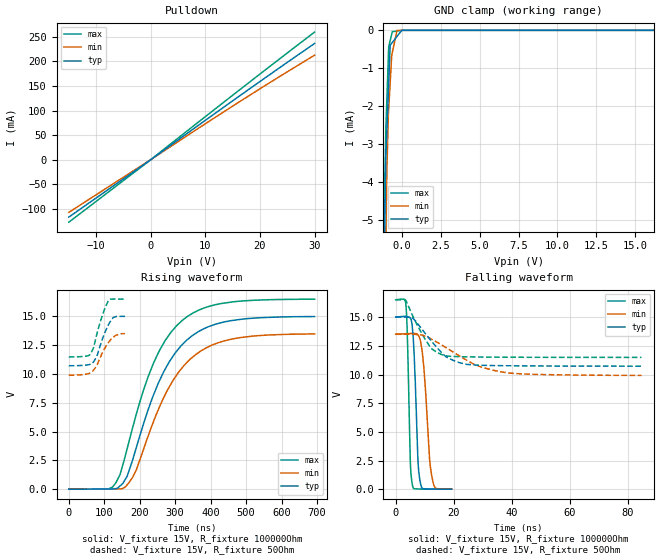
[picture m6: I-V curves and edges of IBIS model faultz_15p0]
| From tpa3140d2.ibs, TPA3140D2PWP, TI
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|   faultz_15p0 Model
[Model]   faultz_15p0
Model_type   Open_drain
Polarity   Non-Inverting
Vmeas = 7.5
Vref = 15
Cref = 2pF
Rref = 100000
|   typ   min   max
|   (nom PVT)   (fast PVT)   (slow PVT)
C_comp   1.652e-13   1.526e-13   1.894e-13
| Where nom  PVT is Nominal Process, 15V, 27C
|   Fast PVT is Strong Process,  16.5V, -40C
|   Slow PVT is Weak Process,   13.5V, 125C
[Voltage Range]   15   13.5   16.5
|Junction Temperature
[Temperature Range]   27   125   -40
[Pullup Reference]   15   13.5   16.5
[Pulldown Reference]   0   0   0
[Power Clamp Reference]   15   13.5   16.5
[GND Clamp Reference]   0   0   0
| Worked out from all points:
|   slope of the pulldown table from 0 to 2.25 V, typ, clamps not added: 124 ohm
|   GND clamp passes 1 mA (typ) near -0.82 V on its own axis
|   falling waveform, V_fixture 15V, R_fixture 100000Ohm: 20-80 % time 1.29ns typ, 2.03ns min, 919ps max; typ from 15 V to 0.026 V
|   rising waveform, V_fixture 15V, R_fixture 100000Ohm: 20-80 % time 120ns typ, 124ns min, 116ns max; typ from 0.019 V to 15 V
|   falling waveform, V_fixture 15V, R_fixture 50Ohm: 20-80 % time 8.71ns typ, 15.3ns min, 6.48ns max; typ from 15 V to 10.7 V
|   rising waveform, V_fixture 15V, R_fixture 50Ohm: 20-80 % time 30.6ns typ, 36.5ns min, 28ns max; typ from 10.7 V to 15 V
[Pulldown]
|   Voltage   I(typ)   I(min)   I(max)
-15V      -116.5mA   -106.9mA   -126.8mA
0V        0A         0A         0A
15.57V    124.1mA    112.9mA    135.8mA
30V       236.2mA    212.4mA    259.3mA
[GND Clamp]
|   Voltage   I(typ)   I(min)   I(max)
-15V      -1.129A    -780mA     -1.389A
-1.155V   -6.507mA   -9.239mA   -5.398mA
-1.121V   -5.497mA   -7.944mA   -4.25mA
-1.04V    -3.321mA   -5.528mA   -2.547mA
-972mV    -2.601mA   -3.62mA    -1.762mA
-858mV    -1.384mA   -2.064mA   -435.8uA
-765mV    -391.9uA   -1.386mA   -274.5uA
-675mV    -344.9uA   -729.4uA   -118.4uA
-627mV    -319.8uA   -587.6uA   -35.21uA
-324mV    -161.5uA   -1.414uA   -20.17uA
-15mV     0A         -65.47nA   -4.838uA
30V       0A         0A         0A
[POWER Clamp]
|   Voltage   I(typ)   I(min)   I(max)
-15V      0A         0A         0A
0V        0A         0A         0A
30V       0A         0A         0A
[Ramp]
R_load = 100000
|   typ   min   max
dV/dt_r   8.98683/1.20201e-07   8.08586/1.24554e-07   9.8876/1.15684e-07
dV/dt_f   8.98876/1.29126e-09   8.08874/2.02787e-09   9.88868/9.19156e-10
[Falling Waveform]
V_fixture = 15V
V_fixture_min = 13.5V
V_fixture_max = 16.5V
R_fixture = 100000Ohm
|   Time   V(typ)   V(min)   V(max)
0s        15V        13.5V      16.5V
3.485ns   15.06V     13.55V     16.18V
3.949ns   15.02V     13.55V     13.93V
5.121ns   14.87V     13.56V     1.914V
5.993ns   13.38V     13.57V     157.1mV
7.658ns   2.58V      13.44V     43.13mV
8.575ns   484mV      12.85V     37.44mV
11.66ns   37.6mV     2.647V     31.43mV
12.87ns   33.79mV    622.7mV    30.22mV
19.25ns   26.25mV    32.03mV    27.36mV
[Rising Waveform]
V_fixture = 15V
V_fixture_min = 13.5V
V_fixture_max = 16.5V
R_fixture = 100000Ohm
|   Time   V(typ)   V(min)   V(max)
0s        18.63mV    18.29mV    18.76mV
111.5ns   19.07mV    24.84mV    19.12mV
132.8ns   59.54mV    26.09mV    570.7mV
164.5ns   1.137V     382.9mV    3.516V
180.4ns   2.597V     1.053V     5.397V
239.5ns   8.232V     5.928V     10.99V
283.4ns   11.07V     8.883V     13.42V
319.5ns   12.54V     10.53V     14.64V
437.1ns   14.5V      12.86V     16.15V
693.1ns   14.98V     13.48V     16.49V
[Falling Waveform]
V_fixture = 15V
V_fixture_min = 13.5V
V_fixture_max = 16.5V
R_fixture = 50Ohm
|   Time   V(typ)   V(min)   V(max)
0s        15V        13.5V      16.5V
3.553ns   15V        13.5V      16.43V
5.794ns   14.92V     13.5V      15.14V
12.16ns   12.95V     13.1V      12.29V
16.78ns   11.66V     12.42V     11.65V
24.37ns   10.88V     11.25V     11.54V
29.24ns   10.81V     10.67V     11.52V
35.87ns   10.77V     10.24V     11.51V
48.13ns   10.74V     10.01V     11.5V
84.61ns   10.72V     9.919V     11.49V
[Rising Waveform]
V_fixture = 15V
V_fixture_min = 13.5V
V_fixture_max = 16.5V
R_fixture = 50Ohm
|   Time   V(typ)   V(min)   V(max)
0s        10.72V     9.89V      11.48V
47.12ns   10.77V     9.98V      11.54V
59.95ns   10.84V     10.09V     11.7V
69.91ns   11.07V     10.35V     12.3V
80.46ns   11.66V     10.84V     13.63V
95.15ns   13.07V     11.86V     15.13V
112.3ns   14.3V      12.76V     16.41V
125.6ns   14.91V     13.19V     16.5V
131.8ns   14.97V     13.35V     16.5V
158.5ns   15V        13.5V      16.5V
